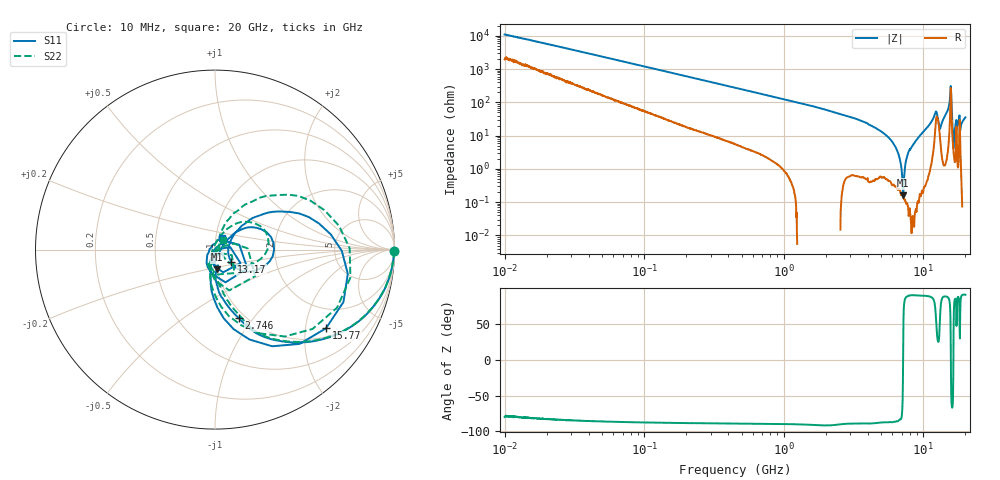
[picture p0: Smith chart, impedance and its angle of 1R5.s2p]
!Keysight Technologies,P5008B,MY61100088,A.16.20.02
!Date: Monday, October 30, 2023 16:17:12
!Correction: S11(C  2-Port  )
!S21(C  2-Port  )
!S12(C  2-Port  )
!S22(C  2-Port  )
!S2P File: Measurements: S11, S21, S12, S22:Log Frequency Sweep
# Hz S  dB  R 50
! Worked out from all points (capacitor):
!   1601 points, 10 MHz to 20 GHz, reference 50 ohm
!   read as one part in series: C = 1.43 pF near 10.39 MHz
!   lowest |Z| = 163 mohm at 7.168 GHz (marker M1)
!   series resonance near 7.157 GHz, so ESL is about 350 pH
!   S11 on the Smith chart (normalised r, x): 10 MHz: open; 2.746 GHz: 0.93, -0.85; 13.17 GHz: 1.19, -0.16; 15.77 GHz: 1.26, -2.60; 20 GHz: 1.07, +0.14
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1e7  -0.01 -0.5  -40.88 79.2  -40.90 79.1  -0.01 -0.5
3.555162e7  -0.03 -1.8  -30.44 83.4  -30.45 83.4  -0.03 -1.8
1.263918e8  -0.08 -6.1  -19.75 81.7  -19.76 81.7  -0.08 -6.1
4.472136e8  -0.59 -20.4  -9.45 68.6  -9.46 68.6  -0.59 -20.2
1.589917e9  -4.02 -54.3  -2.11 36.8  -2.11 36.8  -4.03 -53.8
2.745591e9  -7.86 -70.8  -0.83 19.7  -0.83 19.7  -7.93 -69.0
5.652411e9  -15.43 -88.4  -0.15 0.1  -0.15 0.1  -15.47 -87.2
7.167884e9  -19.08 -84.7  -0.05 -6.3  -0.06 -6.3  -19.17 -105.2
9.264046e9  -22.71 -91.8  -0.00 -14.5  -0.01 -14.6  -23.03 -111.6
1.053187e10  -30.91 -28.4  -0.00 -20.1  -0.01 -20.1  -36.98 -171.0
1.088799e10  -27.94 15.8  -0.02 -22.0  -0.03 -22.0  -32.50 95.3
1.214507e10  -10.97 23.4  -1.38 -34.4  -1.38 -34.5  -11.54 33.7
1.255573e10  -10.52 -16.4  -2.73 -22.5  -2.74 -22.5  -11.65 -11.1
1.316659e10  -18.97 -36.8  -0.69 -18.0  -0.70 -18.1  -24.95 -38.1
1.374174e10  -18.29 35.8  -0.16 -26.3  -0.16 -26.3  -18.59 70.1
1.489756e10  -8.85 34.8  -0.79 -42.4  -0.80 -42.4  -8.84 50.5
1.577149e10  -2.41 -35.3  -11.61 -2.7  -11.61 -2.8  -2.46 -25.5
1.630478e10  -11.32 -91.5  -0.81 -9.6  -0.81 -9.6  -11.43 -88.5
1.726126e10  -15.86 -28.0  -1.68 -26.8  -1.68 -26.9  -15.37 -50.2
1.792989e10  -28.13 45.3  -0.31 -34.3  -0.31 -34.3  -24.22 20.3
1.925417e10  -31.98 163.5  -0.06 -35.1  -0.07 -35.1  -37.54 -110.7
2e10  -22.60 59.2  -0.04 -39.7  -0.04 -39.7  -23.00 49.2
